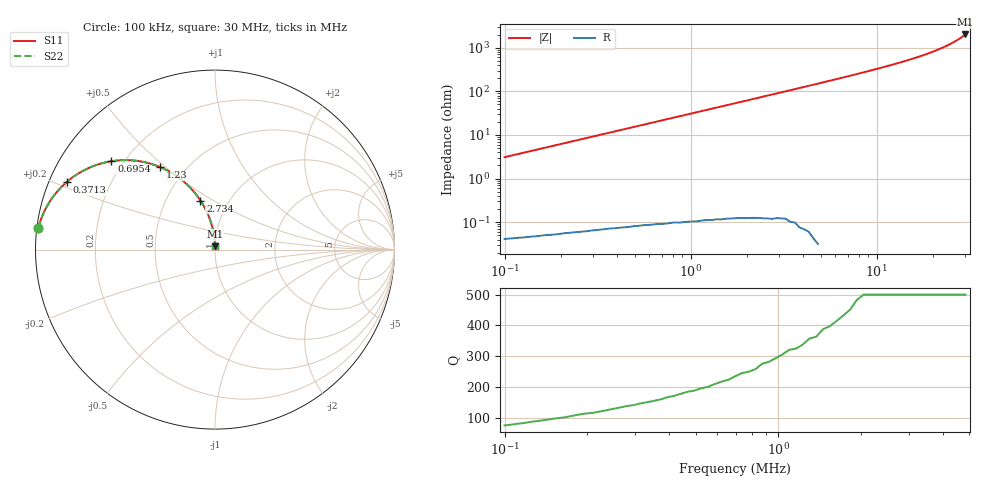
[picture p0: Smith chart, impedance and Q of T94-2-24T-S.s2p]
! ListType=Log
!!T94-2 24T Shunt 2-Port
# MHZ S RI R 50
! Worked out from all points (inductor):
!   101 points, 100 kHz to 30 MHz, reference 50 ohm
!   read as one part in shunt: L = 4.92 uH near 100 kHz
!   highest |Z| = 2.01 kohm at 30 MHz (marker M1)
!   S11 on the Smith chart (normalised r, x): 100 kHz: 0.00, +0.06; 371.3 kHz: 0.05, +0.22; 695.4 kHz: 0.16, +0.36; 1.23 MHz: 0.36, +0.48; 2.734 MHz: 0.74, +0.44; 30 MHz: 1.00, +0.04
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0.1  -0.9839 0.1216  0.0167 0.1215  0.0167 0.1215  -0.9838 0.1216
0.1330014  -0.9724 0.1597  0.028 0.1595  0.028 0.1596  -0.9724 0.1597
0.1768936  -0.9531 0.208  0.0474 0.2077  0.0474 0.2078  -0.953 0.208
0.2637003  -0.9028 0.2933  0.0976 0.2929  0.0976 0.2929  -0.9028 0.2933
0.3713111  -0.8255 0.377  0.1749 0.3765  0.1749 0.3765  -0.8255 0.377
0.4938487  -0.729 0.4423  0.2712 0.4417  0.2712 0.4417  -0.729 0.4423
0.5860135  -0.657 0.4728  0.3431 0.472  0.3431 0.472  -0.657 0.4728
0.6953784  -0.5769 0.4924  0.4232 0.4915  0.4232 0.4916  -0.5769 0.4924
0.9248628  -0.4359 0.4946  0.5639 0.4936  0.5639 0.4936  -0.4359 0.4946
1.23008  -0.3044 0.4593  0.6952 0.4581  0.6952 0.4582  -0.3044 0.4592
1.545319  -0.2171 0.4117  0.7823 0.4105  0.7824 0.4106  -0.2171 0.4117
1.833715  -0.1645 0.3705  0.8349 0.3692  0.8349 0.3692  -0.1645 0.3705
2.175933  -0.1225 0.3279  0.8768 0.3265  0.8768 0.3266  -0.1225 0.3279
2.733571  -0.0809 0.2733  0.9183 0.2717  0.9183 0.2718  -0.0809 0.2733
3.434118  -0.0524 0.2241  0.9467 0.2223  0.9467 0.2223  -0.0524 0.2241
4.567423  -0.0297 0.1721  0.9693 0.1699  0.9693 0.1699  -0.0297 0.1721
7.208434  -0.0113 0.11  0.9877 0.1067  0.9877 0.1067  -0.0113 0.11
12.04431  -0.00311 0.0643  0.9958 0.059  0.9958 0.059  -0.0031 0.0643
16.95935  -0.000865 0.0434  0.9981 0.0361  0.9981 0.0361  -0.000824 0.0434
20.12439  -0.00019 0.035  0.9987 0.0263  0.9987 0.0263  -0.000206 0.035
25.28178  0.000288 0.0252  0.9992 0.0144  0.9992 0.0144  0.00029 0.0252
30  0.000508 0.0188  0.9993 0.00601  0.9993 0.00603  0.00053 0.0188
